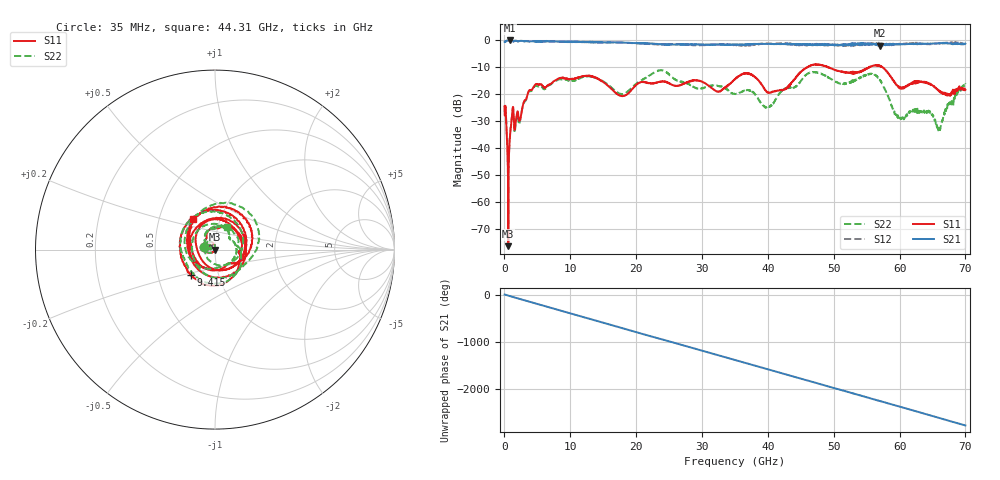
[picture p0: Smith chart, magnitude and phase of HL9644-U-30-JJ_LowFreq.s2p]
! 2/18/2021 8:11:27 AM
! H:\PRODUCTION_DATA\TEMP_S2P.S2P
! CHANNEL.1
! TR.MEASUREMENT
! CORRECTED.DATA
# GHZ S RI R 50.0
! FREQ.GHZ  S11RE  S11IM  S21RE  S21IM  S12RE  S12IM  S22RE  S22IM
!; PortSelection: Port_12
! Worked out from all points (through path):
!   2000 points, 35 MHz to 70 GHz, reference 50 ohm
!   highest |S21| = -0.08 dB at 910 MHz (marker M1); lowest = -2.0 dB at 57.02 GHz (marker M2)
!   group delay of S21, straight-line fit = 109 ps
!   lowest |S11| = -76.2 dB at 595 MHz (marker M3), VSWR 1.00, Z = 50 - j0.0146 ohm
!   |S11| at or under -10 dB: start of sweep to 45.95 GHz; 49.25 GHz to 55.36 GHz (6.108 GHz wide, 11.7 % of centre); 57.41 GHz to end of sweep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
!   |S22| runs from -69.2 to -11.0 dB; largest |S21 - S12| = 0.13
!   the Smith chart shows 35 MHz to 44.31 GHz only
!   S11 on the Smith chart (normalised r, x): 35 MHz: 0.89, +0.02; 9.415 GHz: 0.73, -0.22; 44.31 GHz: 0.75, +0.26
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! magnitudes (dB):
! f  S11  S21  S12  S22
! 35 MHz  -24.4  -0.6  -0.6  -24.3
! 595 MHz  -76.2  -0.1  -0.1  -69.2
! 910 MHz  -33.9  -0.1  -0.1  -33.8
! 1.155 GHz  -28.1  -0.2  -0.2  -28.2
! 2.415 GHz  -29.2  -0.2  -0.2  -29.7
! 3.885 GHz  -18.4  -0.5  -0.5  -18.8
! 9.415 GHz  -14.1  -0.6  -0.5  -14.5
! 11.72 GHz  -13.4  -0.6  -0.6  -13.7
! 17.92 GHz  -20.7  -0.8  -0.9  -19.9
! 23.38 GHz  -15.5  -1.4  -1.6  -11.2
! 32.52 GHz  -19.0  -1.5  -1.4  -16.9
! 35.03 GHz  -14.3  -1.6  -1.6  -19.9
! 37.34 GHz  -12.4  -1.4  -1.6  -18.6
! 39.94 GHz  -19.3  -1.4  -1.2  -24.8
! 44.31 GHz  -13.7  -1.4  -1.4  -17.0
! 46.69 GHz  -9.2  -1.6  -1.6  -11.9
! 57.02 GHz  -9.6  -2.0  -1.1  -14.8
! 58.34 GHz  -12.5  -1.6  -1.3  -21.2
! 59.92 GHz  -17.5  -1.5  -1.4  -28.3
! 64.4 GHz  -15.9  -1.3  -1.4  -26.0
! 65.97 GHz  -18.5  -1.1  -1.2  -32.5
! 70 GHz  -18.3  -1.3  -1.5  -16.2
